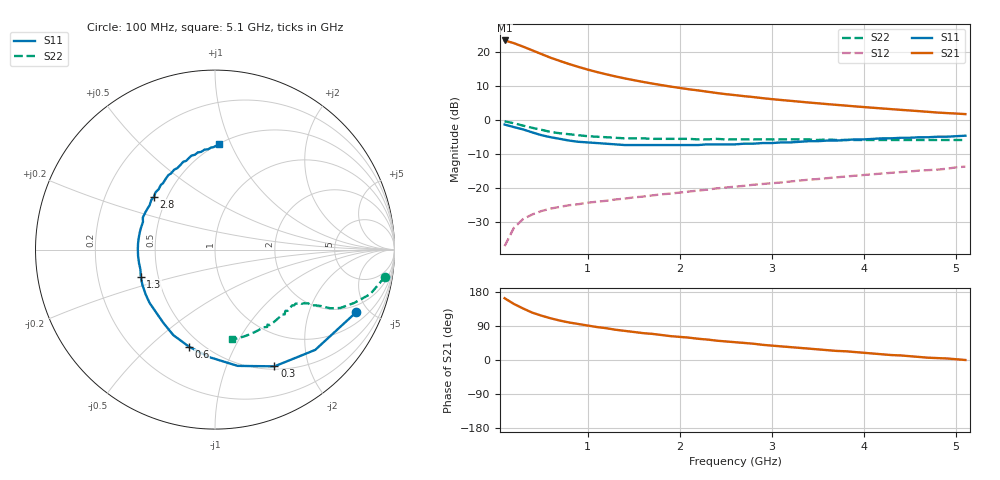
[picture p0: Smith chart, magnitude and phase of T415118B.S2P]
!AT-41511
!S AND NOISE PARAMETERS at Vce=8V  Ic=5mA.  LAST UPDATED 08-03-92
# ghz s ma r 50
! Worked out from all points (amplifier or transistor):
!   51 points, 100 MHz to 5.1 GHz, reference 50 ohm
!   highest |S21| = 23.4 dB at 100 MHz (marker M1)
!   |S21| within 3 dB of that: start of sweep to 408.6 MHz
!   unconditionally stable (mu >= 1): 1.626 GHz to 3.84 GHz
!   at 900 MHz: K = 0.71, MSG = 20.2 dB, |S12| = -24.7 dB
!   at 2.6 GHz: K = 1.10, MAG = 11.6 dB, |S12| = -19.6 dB
!   at 5.1 GHz: K = 0.83, MSG = 7.7 dB, |S12| = -13.7 dB
!   lowest NFmin = 0.90 dB at 100 MHz
!   S11 on the Smith chart (normalised r, x): 100 MHz: 1.55, -4.16; 300 MHz: 0.54, -1.50; 600 MHz: 0.43, -0.67; 1.3 GHz: 0.40, -0.15; 2.8 GHz: 0.42, +0.31; 5.1 GHz: 0.50, +0.90
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0.1  0.86 -24.0  14.84 163.0  0.014 77.0  0.96 -9.0
0.2  0.79 -45.0  13.55 148.0  0.026 67.0  0.9 -16.0
0.3  0.73 -63.0  12.04 136.0  0.035 60.0  0.83 -21.0
0.4  0.66 -79.0  10.62 125.0  0.041 54.0  0.77 -25.0
0.5  0.6 -93.0  9.36 117.0  0.046 51.0  0.72 -27.0
0.6  0.56 -105.0  8.258 110.0  0.05 48.0  0.67 -28.0
0.7  0.53 -116.0  7.412 104.0  0.053 47.0  0.64 -29.0
0.8  0.5 -125.0  6.676 99.0  0.056 46.0  0.62 -30.0
0.9  0.48 -133.0  6.065 95.0  0.058 46.0  0.6 -30.0
1  0.47 -141.0  5.545 91.0  0.061 46.0  0.58 -31.0
1.1  0.46 -147.0  5.101 87.0  0.063 46.0  0.57 -32.0
1.3  0.44 -160.0  4.4 80.0  0.068 47.0  0.55 -33.0
1.6  0.43 -175.0  3.648 71.0  0.075 48.0  0.54 -35.0
1.8  0.43 176.0  3.274 66.0  0.081 49.0  0.53 -37.0
2.2  0.43 159.0  2.735 56.0  0.092 50.0  0.52 -41.0
2.4  0.44 152.0  2.507 51.0  0.099 51.0  0.53 -43.0
2.6  0.44 146.0  2.33 47.0  0.105 51.0  0.52 -45.0
2.8  0.45 139.0  2.182 43.0  0.112 51.0  0.52 -47.0
3  0.46 133.0  2.035 38.0  0.118 51.0  0.52 -49.0
3.5  0.49 120.0  1.766 28.0  0.136 50.0  0.51 -55.0
4.3  0.54 102.0  1.449 13.0  0.168 48.0  0.51 -66.0
5.1  0.59 88.0  1.226 0.0  0.207 45.0  0.51 -79.0
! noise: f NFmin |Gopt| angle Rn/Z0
0.1  0.9  0.6  6  0.29
0.9  1.1  0.48  57  0.22
1.8  1.4  0.35  124  0.14
2.4  1.6  0.4  167  0.09
